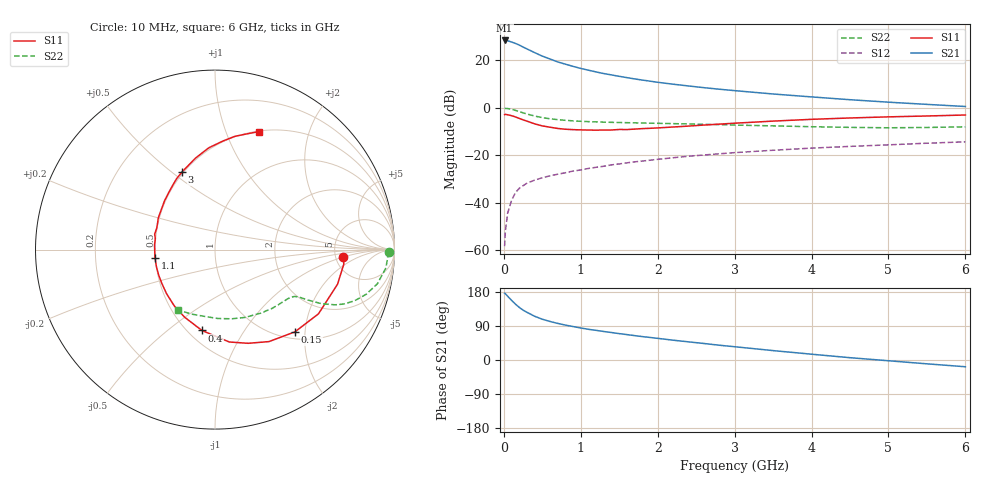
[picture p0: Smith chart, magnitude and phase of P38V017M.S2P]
! SIEMENS Small Signal Semiconductors
! BFP181
! Si NPN RF Bipolar Junction Transistor in SOT143
! VCE = 8 V  IC = 17 mA
! Common Emitter S-Parameters:  March  1996
# GHz  S  MA  R  50
!  f  S11  S21  S12  S22
! GHz  MAG  ANG  MAG  ANG  MAG  ANG  MAG  ANG
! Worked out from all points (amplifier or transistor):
!   36 points, 10 MHz to 6 GHz, reference 50 ohm
!   highest |S21| = 28.4 dB at 10 MHz (marker M1)
!   |S21| within 3 dB of that: start of sweep to 263.9 MHz
!   unconditionally stable (mu >= 1): 997.1 MHz to end of sweep
!   at 250 MHz: K = 0.41, MSG = 29.2 dB, |S12| = -32.9 dB
!   at 1.4 GHz: K = 1.09, MAG = 17.1 dB, |S12| = -24.1 dB
!   at 6 GHz: K = 1.00, MAG = 7.1 dB, |S12| = -14.4 dB
!   S11 on the Smith chart (normalised r, x): 10 MHz: 5.85, -0.92; 150 MHz: 1.14, -1.77; 400 MHz: 0.58, -0.67; 1.1 GHz: 0.50, -0.05; 3 GHz: 0.49, +0.55; 6 GHz: 0.51, +1.31
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0.01  0.7142 -3.1  26.17 176.4  0.0012 69.5  0.9673 -0.8
0.02  0.7224 -6.4  26.03 175.0  0.0025 80.4  0.9637 -2.2
0.05  0.7094 -15.8  25.69 168.2  0.006 85.6  0.9577 -6.1
0.1  0.6786 -31.8  24.28 157.6  0.0111 73.7  0.9245 -11.9
0.15  0.6391 -45.8  22.69 147.6  0.016 68.6  0.8779 -16.5
0.2  0.5943 -59.6  20.96 138.9  0.0199 63.9  0.8275 -20.2
0.25  0.5538 -70.5  19 131.6  0.0226 61.1  0.779 -22.9
0.3  0.5209 -81.2  17.37 125.9  0.0256 57.7  0.7364 -24.7
0.4  0.4563 -99.2  14.51 115.4  0.0296 55.4  0.6669 -26.9
0.5  0.413 -114.2  12.22 107.6  0.0333 53.4  0.6173 -27.9
0.6  0.3873 -125.8  10.63 101.7  0.0366 52.8  0.5834 -28.6
0.7  0.3648 -137.8  9.236 96.6  0.0395 52.8  0.5591 -29.0
0.9  0.3444 -155.7  7.437 88.3  0.0461 53.1  0.5269 -29.9
1.1  0.3373 -171.9  6.178 81.0  0.0523 53.2  0.5079 -31.1
1.3  0.3379 175.5  5.242 75.2  0.0582 53.2  0.4955 -32.8
1.6  0.3457 160.1  4.306 67.0  0.0686 52.1  0.483 -35.9
2.2  0.3912 135.9  3.129 52.3  0.0879 49.2  0.4606 -43.9
3  0.4705 112.9  2.289 35.0  0.1127 43.3  0.4294 -56.7
3.5  0.5209 102.1  1.944 24.8  0.1265 39.4  0.4134 -66.1
4.5  0.6067 85.8  1.473 6.1  0.1526 31.0  0.3843 -87.6
5.5  0.6681 74.7  1.174 -10.1  0.1782 23.7  0.3825 -110.2
6  0.7009 69.7  1.059 -17.8  0.1904 19.6  0.3946 -121.9
